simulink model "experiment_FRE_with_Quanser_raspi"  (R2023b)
settings: configuration reference "FRE_experiment_config_PIL" (kept in a data dictionary, not in this file)
libraries: simulink x2

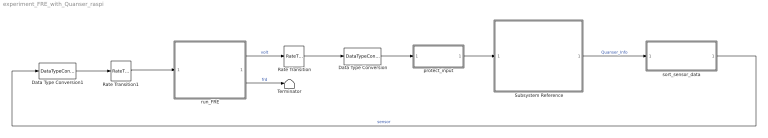
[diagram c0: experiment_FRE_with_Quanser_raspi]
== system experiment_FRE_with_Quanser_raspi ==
  Data Type Conversion : DataTypeConversion  OutDataTypeStr=double
  Data Type Conversion1 : DataTypeConversion  OutDataTypeStr=single
  Rate Transition : RateTransition
  Rate Transition1 : RateTransition  OutPortSampleTime=FRE_time_step
  Subsystem Reference : Subsystem  ReferencedSubsystem=raspi_Quanser
  Terminator : Terminator
  protect_input : Subsystem  ReferencedSubsystem=protect_input
  run_FRE : ModelReference  ModelNameDialog=run_FRE.slx  SimulationMode=Normal  ModelReferenceVersion=1.29
  sort_sensor_data : Subsystem
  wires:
  Rate Transition/1 -> Data Type Conversion/1
  Rate Transition1/1 -> run_FRE/1
  Data Type Conversion1/1 -> Rate Transition1/1
  run_FRE/1 -> Rate Transition/1  "volt"
  run_FRE/2 -> Terminator/1  "frd"
  Data Type Conversion/1 -> protect_input/1
  sort_sensor_data/1(sensor) -> Data Type Conversion1/1  "sensor"
  Subsystem Reference/1 -> sort_sensor_data/1(Quanser_Info)  "Quanser_Info"
  protect_input/1 -> Subsystem Reference/1

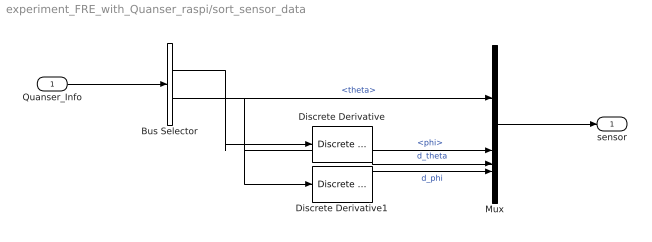
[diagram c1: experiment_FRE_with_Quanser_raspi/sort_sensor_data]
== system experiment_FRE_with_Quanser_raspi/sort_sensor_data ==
  Quanser_Info : Inport
  Bus Selector : BusSelector  OutputSignals=theta,phi
  Discrete Derivative : simulink/Discrete/Discrete Derivative  gainval=1.0  ICPrevScaledInput=0.0  OutMin=[]  OutMax=[]  OutDataType=fixdt(1, 16)  OutScaling=2^-10  DoSatur=off
  Discrete Derivative1 : simulink/Discrete/Discrete Derivative  gainval=1.0  ICPrevScaledInput=0.0  OutMin=[]  OutMax=[]  OutDataType=fixdt(1, 16)  OutScaling=2^-10  DoSatur=off
  Mux : Mux
  sensor : Outport
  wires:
  Quanser_Info/1 -> Bus Selector/1
  Bus Selector/1 -> Discrete Derivative/1, Mux/1  "<theta>"
  Bus Selector/2 -> Discrete Derivative1/1, Mux/2  "<phi>"
  Discrete Derivative1/1 -> Mux/4  "d_phi"
  Mux/1 -> sensor/1
  Discrete Derivative/1 -> Mux/3  "d_theta"
